(* Logix 5000 AddOnInstructionDefinition export Banner_Q4X_PD_v4; software revision 33.00 *)

TYPE Banner_Q4X_PDI_v4 :   // UDT that records the converted prcoess data.
STRUCT
   Channel_1_Output_State : SINT;   // 0 = Inactive, 1 = Active
   Channel_2_Output_State : SINT;   // 0 = Inactive, 1 = Active
   Sensor_Stability : SINT;   // 0 = No target or Marginal signal, 1 = Stable signal
   Measurement_Value : REAL;   // Distance from sensor face in mm's.
END_STRUCT
END_TYPE

ADD_ON_INSTRUCTION Banner_Q4X_PD_v4   (* revision 4.1, vendor Banner Engineering *)
// Takes the raw SINT information and converts that data into actual information.
VAR_IN_OUT
   SINT0 : SINT; {required}
   SINT1 : SINT; {required}
   PROCESS_DATA : Banner_Q4X_PDI_v4; {required}
END_VAR
VAR_INPUT
   Byte_Swap : BOOL; {required}   // Swap the LSB and the MSB with each other.
END_VAR
VAR
   Temp_Measurement : DINT; {access None}
   Data_Byte : SINT[2]; {access None}
END_VAR

ROUTINE Logic   (* ladder *)
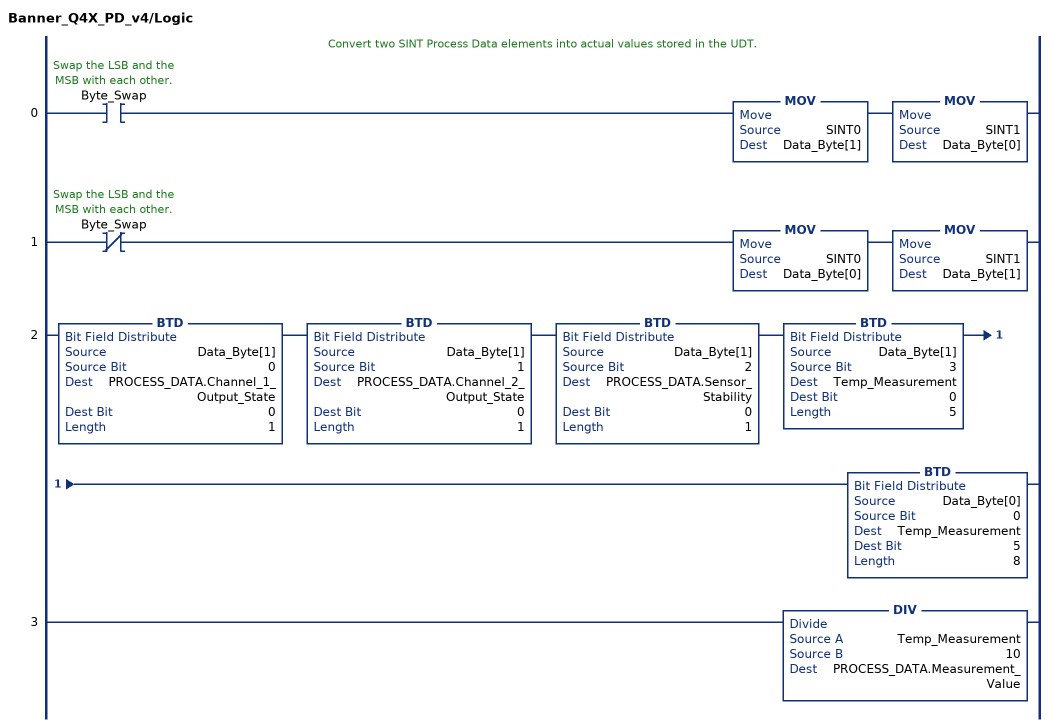
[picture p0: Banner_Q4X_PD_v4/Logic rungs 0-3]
   // Convert two SINT Process Data elements into actual values stored in the UDT.
   0: XIC(Byte_Swap)MOV(SINT0,Data_Byte[1])MOV(SINT1,Data_Byte[0]);
   1: XIO(Byte_Swap)MOV(SINT0,Data_Byte[0])MOV(SINT1,Data_Byte[1]);
   2: BTD(Data_Byte[1],0,PROCESS_DATA.Channel_1_Output_State,0,1)BTD(Data_Byte[1],1,PROCESS_DATA.Channel_2_Output_State,0,1)BTD(Data_Byte[1],2,PROCESS_DATA.Sensor_Stability,0,1)BTD(Data_Byte[1],3,Temp_Measurement,0,5)BTD(Data_Byte[0],0,Temp_Measurement,5,8);
   3: DIV(Temp_Measurement,10,PROCESS_DATA.Measurement_Value);
END_ROUTINE
END_ADD_ON_INSTRUCTION
